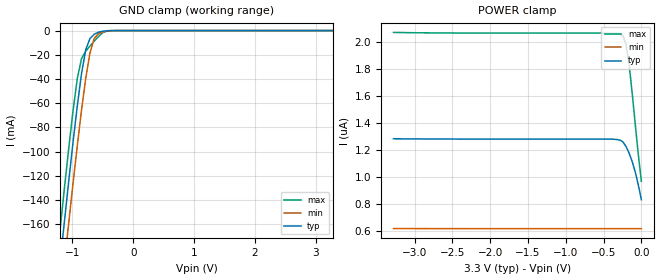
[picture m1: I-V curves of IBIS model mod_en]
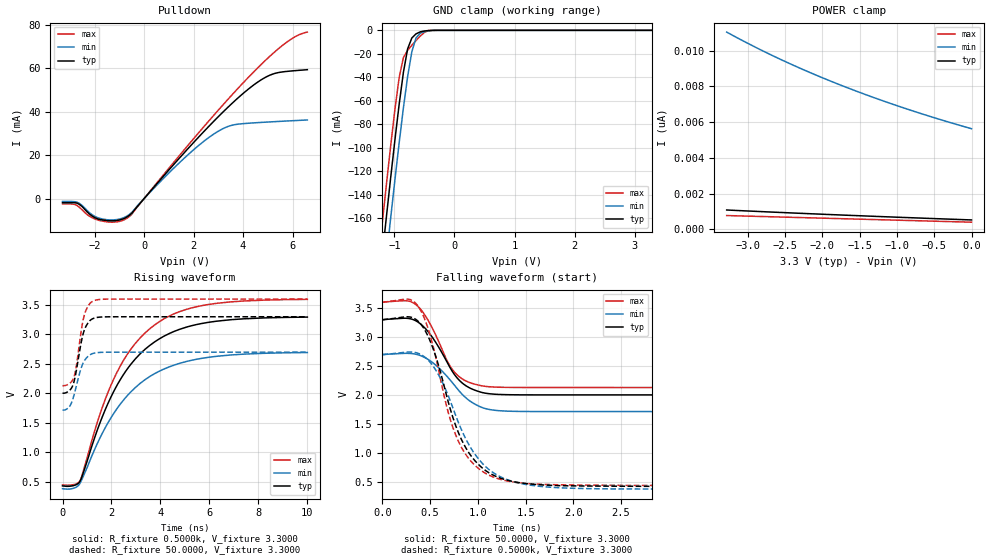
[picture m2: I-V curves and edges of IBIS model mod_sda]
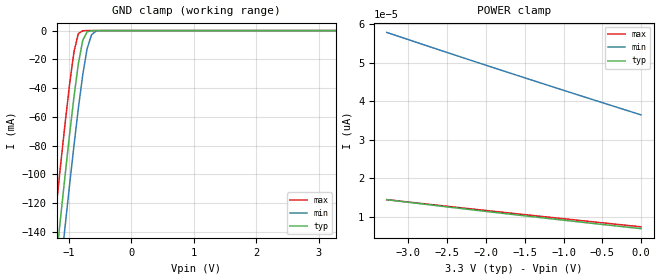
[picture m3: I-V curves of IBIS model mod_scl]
| IBIS (I/O, Buffer, Information, Specification) Model, officially
| electronic behavioral standard for Buffer structures of digital pins.
[IBIS ver]  4.0
[File name] m24c04_fa2_tssop8.ibs
[File Rev]  1.0
[Date]   5 Dic 2014
[Source]   CAD & Design Services (Catania) - STMicroelectronics
[Notes]
   (Note1)  This IBIS model includes the TSSOP8 package data
   (Note2)  This IBIS model has some Notes about the non-monotonicity
   of the I-V curves, but they are not indicative of problems
   inside the model;
[Copyright] (c) 2014 STMicroelectronics
|   Component M24C04
[Component] M24C04
[Manufacturer] STMicroelectronics
[Package]
| variable   typ   min   max
R_pkg   0.0   0.0   0.0
L_pkg   0.0H   0.0H   0.0H
C_pkg   0.0F   0.0F   0.0F
[Pin]  signal_name   model_name   R_pin   L_pin   C_pin
1   NC   NC   NA   NA   NA
2   E1   mod_en   NA   NA   NA
3   E2   mod_en   NA   NA   NA
4   VSS   GND   NA   NA   NA
5   SDA   mod_sda   NA   NA   NA
6   SCL   mod_scl   NA   NA   NA
7   WCN   mod_wc   NA   NA   NA
8   VCC   POWER   NA   NA   NA
[Package Model]  182696_TSSOP8
[Define Package Model]  182696_TSSOP8
[Manufacturer]  STMicroelectronics
[OEM]  STMicroelectronics
[Description]  8 pin TSSOP package
[Number Of Pins]  8
[Pin Numbers]
|Pin Num   Terminal Name
1   | net1
2   | net2
3   | net3
4   | net4_GND
5   | net5
6   | net6
7   | net7
8   | net8_VDD
[Model Data]
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[End Model Data]
[End Package Model]
| Models and submodels in the file (4): mod_en (Input), mod_sda (I/O_open_drain), mod_scl (Input), mod_wc (Input)
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|   Model mod_en
[Model]   mod_en
Model_type Input
Vinl   =   1.000V
Vinh   =   2.300V
C_comp   1.763pF   1.683pF   1.933pF
[Temperature Range]  25.0000   85.0000   -40.0000
[Voltage Range]   3.3000V   2.7000V   3.6000V
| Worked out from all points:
|   GND clamp passes 1 mA (typ) near -0.54 V on its own axis
[GND_clamp]
|Voltage   I(typ)   I(min)   I(max)
-3.3V     -1.254A    -1.285A    -1.23A
-1.27V    -225.1mA   -259.5mA   -197.7mA
-1.2V     -191.1mA   -225.7mA   -163.7mA
-1.13V    -157.7mA   -192.2mA   -130.2mA
-1.06V    -124.9mA   -159.2mA   -97.74mA
-920mV    -62.84mA   -95.74mA   -40.11mA
-850mV    -35.89mA   -66.17mA   -23.29mA
-780mV    -15.88mA   -39.51mA   -17.03mA
-710mV    -6.558mA   -18.36mA   -12.75mA
-640mV    -3.016mA   -6.443mA   -8.697mA
-360mV    -24uA      -153.5uA   -7.885uA
3.28V     528.3pA    6.354nA    369.1pA
[POWER_clamp]
|Voltage   I(typ)   I(min)   I(max)
-3.28V    1.284uA    617.5nA    2.074uA
-400mV    1.282uA    616.6nA    2.069uA
-280mV    1.273uA    616.6nA    2.062uA
-240mV    1.258uA    616.6nA    2.044uA
-200mV    1.223uA    616.6nA    1.977uA
-160mV    1.175uA    616.6nA    1.826uA
-120mV    1.112uA    616.6nA    1.615uA
-80mV     1.036uA    616.6nA    1.388uA
-40mV     940nA      616.5nA    1.165uA
0V        832nA      616.5nA    968.6nA
|   Model mod_sda
[Model]   mod_sda
Model_type I/O_open_drain
Polarity   Non-Inverting
Vinl   =   1.000V
Vinh   =   2.300V
Vmeas  =   1.650V
Cref   =   10pF
Rref   =   1k
Vref   =   3.300V
C_comp   3.856pF   3.682pF   4.038pF
[Temperature Range]  25.0000   85.0000   -40.0000
[Voltage Range]   3.3000V   2.7000V   3.6000V
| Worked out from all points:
|   slope of the pulldown table from 0 to 0.495 V, typ, clamps not added: 75.4 ohm
|   GND clamp passes 1 mA (typ) near -0.54 V on its own axis
|   rising waveform, R_fixture 0.5000k, V_fixture 3.3000: 20-80 % time 2.18ns typ, 2.26ns min, 2.11ns max; typ from 0.432 V to 3.29 V
|   rising waveform, R_fixture 50.0000, V_fixture 3.3000: 20-80 % time 358ps typ, 399ps min, 329ps max; typ from 2.01 V to 3.3 V
|   falling waveform, R_fixture 50.0000, V_fixture 3.3000: 20-80 % time 298ps typ, 336ps min, 268ps max; typ from 3.3 V to 2.01 V
|   falling waveform, R_fixture 0.5000k, V_fixture 3.3000: 20-80 % time 361ps typ, 412ps min, 326ps max; typ from 3.3 V to 0.432 V
[Pulldown]
|Voltage   I(typ)   I(min)   I(max)
-3.3V     -1.866mA   -1.32mA    -2.4mA
-2.7V     -2.162mA   -1.737mA   -3.278mA
-2.2V     -7.236mA   -6.637mA   -8.202mA
-1.8V     -9.611mA   -9.071mA   -10.11mA
-1.2V     -10.21mA   -9.782mA   -10.82mA
-700mV    -8.503mA   -8.075mA   -9.112mA
1.7V      22.07mA    19.4mA     23.51mA
3.1V      38.83mA    31.66mA    42mA
3.7V      45.34mA    34.1mA     49.56mA
4.9V      55.78mA    35.17mA    63.57mA
5.9V      58.69mA    35.78mA    73.06mA
6.6V      59.34mA    36.18mA    76.65mA
[GND_clamp]
|Voltage   I(typ)   I(min)   I(max)
-3.3V     -1.254A    -1.285A    -1.23A
-1.27V    -225.1mA   -259.5mA   -197.7mA
-1.2V     -191.1mA   -225.7mA   -163.7mA
-1.13V    -157.7mA   -192.2mA   -130.2mA
-1.06V    -124.9mA   -159.2mA   -97.74mA
-920mV    -62.84mA   -95.74mA   -40.11mA
-850mV    -35.89mA   -66.17mA   -23.29mA
-780mV    -15.88mA   -39.51mA   -17.03mA
-710mV    -6.558mA   -18.36mA   -12.75mA
-640mV    -3.016mA   -6.443mA   -8.697mA
-360mV    -24uA      -153.5uA   -7.885uA
3.28V     528.3pA    6.354nA    369.1pA
[POWER_clamp]
|Voltage   I(typ)   I(min)   I(max)
-3.28V    1.087nA    11.04nA    776.5pA
-2.92V    1.017nA    10.25nA    735.5pA
-2.56V    950pA      9.515nA    694.5pA
-2.16V    878.3pA    8.77nA     649.1pA
-1.76V    809.4pA    8.084nA    603.8pA
-1.36V    742.9pA    7.453nA    558.6pA
-920mV    672.2pA    6.813nA    508.9pA
-480mV    603.7pA    6.224nA    459.2pA
0V        531.3pA    5.634nA    405.2pA
[Ramp]
| variable   typ   min   max
dV/dt_r   0.7762/0.4137n   0.5882/0.4828n   0.8801/0.3891n
dV/dt_f   0.7762/0.3204n   0.5882/0.3795n   0.8801/0.3032n
R_load = 50.0000
[Rising Waveform]
R_fixture= 0.5000k
V_fixture= 3.3000
V_fixture_min= 2.7000
V_fixture_max= 3.6000
|time   V(typ)   V(min)   V(max)
0s        432.3mV    385.1mV    449.6mV
430ps     435.1mV    389.8mV    451.7mV
730ps     522.7mV    489mV      532.2mV
1.51ns    1.479V     1.228V     1.623V
2.13ns    2.064V     1.685V     2.278V
2.97ns    2.584V     2.099V     2.847V
3.77ns    2.876V     2.338V     3.164V
4.77ns    3.085V     2.509V     3.385V
5.94ns    3.204V     2.611V     3.507V
10ns      3.294V     2.694V     3.595V
[Rising Waveform]
R_fixture= 50.0000
V_fixture= 3.3000
V_fixture_min= 2.7000
V_fixture_max= 3.6000
|time   V(typ)   V(min)   V(max)
0s        2.006V     1.72V      2.133V
270ps     2.045V     1.772V     2.164V
350ps     2.081V     1.826V     2.192V
450ps     2.171V     1.944V     2.258V
550ps     2.356V     2.101V     2.432V
770ps     2.88V      2.441V     3.077V
890ps     3.073V     2.553V     3.327V
1.07ns    3.212V     2.639V     3.498V
1.31ns    3.279V     2.685V     3.576V
10ns      3.3V       2.7V       3.6V
[Falling Waveform]
R_fixture= 50.0000
V_fixture= 3.3000
V_fixture_min= 2.7000
V_fixture_max= 3.6000
|time   V(typ)   V(min)   V(max)
0s        3.3V       2.7V       3.6V
240ps     3.325V     2.721V     3.627V
350ps     3.282V     2.707V     3.561V
430ps     3.183V     2.661V     3.417V
510ps     3.028V     2.582V     3.198V
670ps     2.594V     2.338V     2.621V
750ps     2.368V     2.183V     2.408V
890ps     2.149V     1.935V     2.235V
1.11ns    2.029V     1.759V     2.148V
10ns      2.006V     1.72V      2.133V
[Falling Waveform]
R_fixture= 0.5000k
V_fixture= 3.3000
V_fixture_min= 2.7000
V_fixture_max= 3.6000
|time   V(typ)   V(min)   V(max)
0s        3.3V       2.7V       3.6V
370ps     3.281V     2.724V     3.542V
470ps     3.044V     2.62V      3.191V
570ps     2.614V     2.405V     2.579V
690ps     1.886V     1.992V     1.705V
810ps     1.305V     1.478V     1.163V
1.03ns    773.3mV    859.5mV    711.2mV
1.31ns    538.2mV    547.1mV    525.2mV
2.25ns    437.9mV    392.3mV    452.9mV
10ns      432.3mV    385.1mV    449.6mV
|   Model mod_scl
[Model]   mod_scl
Model_type Input
Vinl   =   1.000V
Vinh   =   2.300V
C_comp   1.763pF   1.683pF   1.933pF
[Temperature Range]  25.0000   85.0000   -40.0000
[Voltage Range]   3.3000V   2.7000V   3.6000V
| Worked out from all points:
|   GND clamp passes 1 mA (typ) near -0.71 V on its own axis
[GND_clamp]
|Voltage   I(typ)   I(min)   I(max)
-3.3V     -1.086A    -1.119A    -1.052A
-1.27V    -186.8mA   -222.8mA   -150.3mA
-1.2V     -157.3mA   -193.3mA   -120.7mA
-1.13V    -128.1mA   -164mA     -91.65mA
-1.06V    -99.56mA   -135.2mA   -63.53mA
-920mV    -45.89mA   -79.74mA   -14.62mA
-850mV    -22.95mA   -53.94mA   -2.113mA
-780mV    -6.754mA   -30.77mA   -106.4uA
-710mV    -883.8uA   -12.62mA   -4.426uA
-640mV    -77.7uA    -2.974mA   -182.3nA
-570mV    -6.449uA   -439.9uA   -7.506nA
3.28V     6.813pA    40.1pA     6.666pA
[POWER_clamp]
|Voltage   I(typ)   I(min)   I(max)
-3.28V    14.38pA    57.84pA    14.39pA
-2.52V    12.55pA    52.74pA    12.71pA
-1.72V    10.69pA    47.47pA    10.97pA
0V        6.856pA    36.42pA    7.331pA
